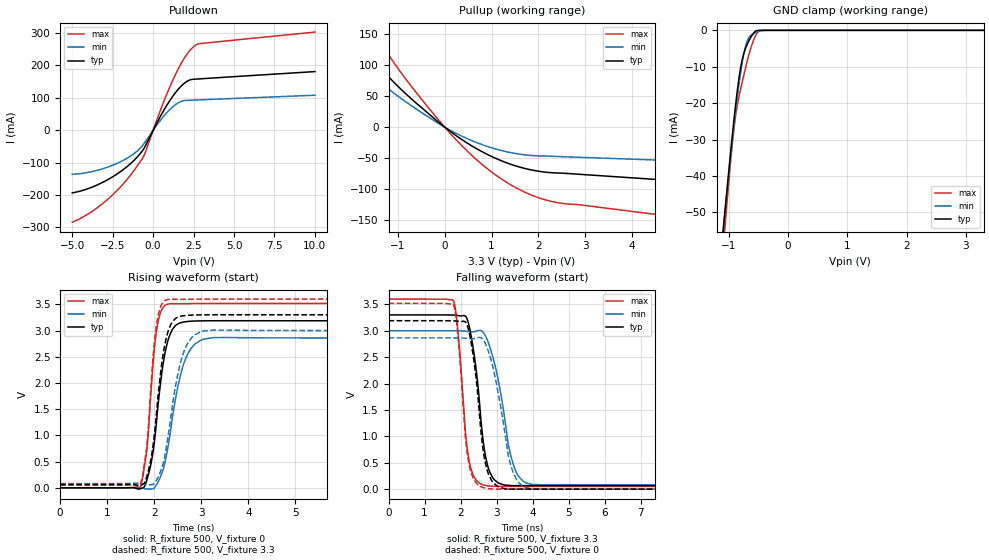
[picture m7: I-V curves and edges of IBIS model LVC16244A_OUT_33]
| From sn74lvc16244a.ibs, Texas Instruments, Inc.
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[Model]   LVC16244A_OUT_33
Model_type  3-state
Enable   Active-Low
Vref =   0
Rref =   500
Cref =   50p
Vmeas =   1.5
| variable   typ   min   max
C_comp   4.66pF   4.13pF   6.00pF
| C_pullup   6.54pF   3.89pF   9.70pF
| C_pulldown   6.87pF   5.28pF   8.79pF
| C_tri-state   4.66pF   4.13pF   6.00pF
[Temperature Range]   40   100   -40
| Ambient temperature   25   85   -40
[Voltage range]   3.3   3   3.6
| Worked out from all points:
|   slope of the pulldown table from 0 to 0.495 V, typ, clamps not added: 10.5 ohm
|   slope of the pullup table from 0 to 0.495 V, typ, clamps not added: 18.7 ohm
|   GND clamp passes 1 mA (typ) near -0.59 V on its own axis
|   rising waveform, R_fixture 500, V_fixture 0: 20-80 % time 259ps typ, 351ps min, 182ps max; typ from 0 V to 3.19 V
|   falling waveform, R_fixture 500, V_fixture 3.3: 20-80 % time 316ps typ, 456ps min, 245ps max; typ from 3.3 V to 0.065 V
|   rising waveform, R_fixture 500, V_fixture 3.3: 20-80 % time 249ps typ, 331ps min, 179ps max; typ from 0.065 V to 3.3 V
|   falling waveform, R_fixture 500, V_fixture 0: 20-80 % time 305ps typ, 442ps min, 241ps max; typ from 3.19 V to 0 V
[GND Clamp]
| LVC16244A_OUT_33
|   Voltage   I(typ)   I(min)   I(max)
-5V       -855.7mA   -797.6mA   -953.2mA
-1.095V   -55.25mA   -54.79mA   -60.22mA
-1.065V   -49.94mA   -49.9mA    -54.27mA
-955mV    -31.29mA   -32.66mA   -33.81mA
-910mV    -24.24mA   -26.03mA   -26.76mA
-860mV    -17.12mA   -19.11mA   -20.92mA
-795mV    -9.817mA   -11.17mA   -15.81mA
-735mV    -5.784mA   -5.591mA   -11.55mA
-680mV    -3.534mA   -2.583mA   -7.881mA
-580mV    -736.5uA   -852.5uA   -2.652mA
-485mV    -14.03uA   -258.5uA   -126.7uA
3.3V      10.95pA    55.96nA    -30.28pA
[Pulldown]
| LVC16244A_OUT_33
|   Voltage   I(typ)   I(min)   I(max)
-5V       -193.4mA   -135.8mA   -283.8mA
-3.87V    -177.4mA   -128.6mA   -253.7mA
-2.72V    -150.1mA   -112.1mA   -209.2mA
-1.54V    -109.1mA   -84.13mA   -147.4mA
-730mV    -67.77mA   -51.47mA   -92.05mA
-485mV    -48.43mA   -35.35mA   -68.52mA
485mV     46.17mA    33.18mA    66.28mA
1.245V    107.2mA    73.64mA    157.8mA
1.945V    145.9mA    91.78mA    224mA
2.535V    157.6mA    93.17mA    259.6mA
2.87V     158.7mA    93.86mA    267.5mA
10V       181.2mA    108.1mA    303.1mA
[Pullup]
| LVC16244A_OUT_33
|   Voltage   I(typ)   I(min)   I(max)
-5V       388.2mA    115.6mA    569.5mA
-4.8V     377.1mA    131.8mA    547.8mA
-4.67V    368.8mA    170.1mA    533.4mA
-2.73V    213.4mA    164.5mA    302.6mA
-2.425V   186.8mA    144.1mA    265.2mA
-1.63V    117.9mA    90.44mA    167.3mA
-735mV    47.21mA    35.83mA    68.13mA
480mV     -25.67mA   -18.52mA   -38.57mA
1.275V    -56.24mA   -38.95mA   -86.83mA
2.13V     -72.49mA   -46.66mA   -117mA
6.525V    -94.6mA    -58.57mA   -160mA
10V       -112.3mA   -68.03mA   -193.4mA
[Ramp]
| LVC16244A_OUT_33
| variable   typ   min   max
dV/dt_r   1.93/2.68E-10   1.73/3.64E-10   2.13/1.89E-10
dV/dt_f   1.94/3.22E-10   1.76/4.75E-10   2.13/2.54E-10
R_load = 500
[Rising Waveform]
| LVC16244A_OUT_33
R_fixture =   500
C_fixture =   0
L_fixture =   0
V_fixture =   0
V_fixture_min = 0
V_fixture_max = 0
|   Time   V(typ)   V(min)   V(max)
0s        164.3pV    3.691nV    4.973nV
1.71ns    -16.36mV   1.551mV    34.15mV
1.845ns   158mV      -21.95mV   747.5mV
1.975ns   697.1mV    -19.75mV   2.392V
2.055ns   1.335V     68.45mV    3.038V
2.18ns    2.317V     325.8mV    3.428V
2.32ns    2.89V      935.7mV    3.51V
2.685ns   3.171V     2.503V     3.513V
3.275ns   3.187V     2.866V     3.517V
50ns      3.186V     2.859V     3.517V
[Falling Waveform]
| LVC16244A_OUT_33
R_fixture =   500
C_fixture =   0
L_fixture =   0
V_fixture =   3.3
V_fixture_min = 3
V_fixture_max = 3.6
|   Time   V(typ)   V(min)   V(max)
0s        3.3V       3V         3.6V
1.805ns   3.296V     3V         3.561V
1.94ns    3.287V     2.999V     2.904V
2.15ns    3.268V     2.991V     983.3mV
2.365ns   2.604V     2.98V      245.4mV
2.64ns    851.8mV    2.961V     79.23mV
2.81ns    327.2mV    2.701V     57.49mV
3.46ns    65.56mV    479.7mV    50.51mV
4.015ns   65.55mV    86.54mV    50.17mV
50ns      65.09mV    80.64mV    50.19mV
[Rising Waveform]
| LVC16244A_OUT_33
R_fixture =   500
C_fixture =   0
L_fixture =   0
V_fixture =   3.3
V_fixture_min = 3
V_fixture_max = 3.6
|   Time   V(typ)   V(min)   V(max)
0s        65.06mV    80.58mV    50.18mV
1.71ns    49.29mV    81.62mV    85.45mV
1.845ns   229.7mV    58.66mV    821.7mV
1.975ns   817.8mV    64.07mV    2.516V
2.055ns   1.506V     158mV      3.156V
2.18ns    2.502V     438.3mV    3.526V
2.315ns   3.038V     1.117V     3.596V
2.67ns    3.287V     2.684V     3.596V
3.25ns    3.3V       3.009V     3.6V
50ns      3.3V       3V         3.6V
[Falling Waveform]
| LVC16244A_OUT_33
R_fixture =   500
C_fixture =   0
L_fixture =   0
V_fixture =   0
V_fixture_min = 0
V_fixture_max = 0
|   Time   V(typ)   V(min)   V(max)
0s        3.19V      2.864V     3.519V
1.8ns     3.187V     2.864V     3.487V
1.935ns   3.179V     2.863V     2.849V
2.145ns   3.162V     2.856V     916.6mV
2.365ns   2.458V     2.848V     188mV
2.62ns    774.9mV    2.835V     31.65mV
2.81ns    234.5mV    2.534V     6.652mV
3.415ns   -277uV     406.7mV    356.9uV
3.995ns   237.6uV    5.6mV      5.493uV
50ns      28.28uV    54.73uV    9.888uV
